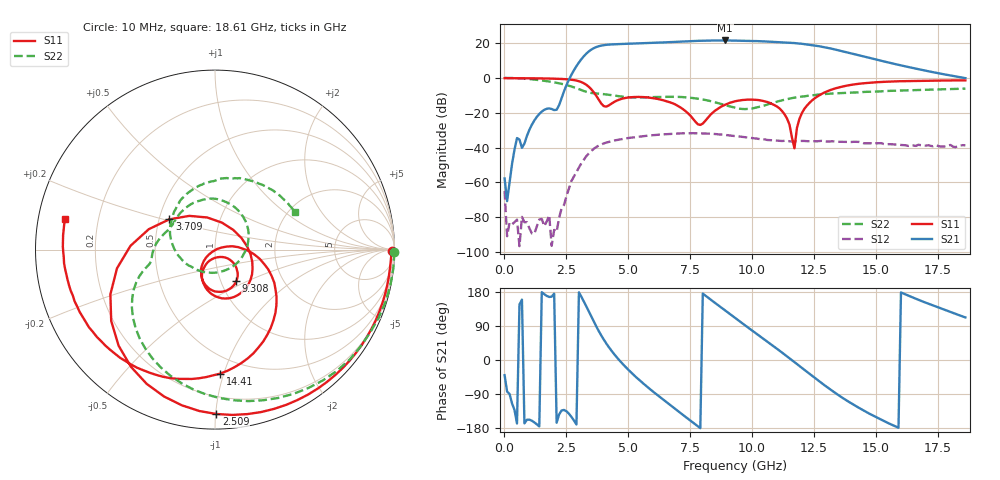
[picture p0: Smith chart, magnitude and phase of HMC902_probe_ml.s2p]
! Hittite Microwave Corporation
! 20 Alpha Road
! Chelmsford, MA 01824
! http://www.hittite.com
! Tel: 978-250-3343
! Fax: 978-250-3373
! Device:  HMC902
! Description: GaAs HEMT MMIC Low Noise Amplifier
! Frequency:  5.00 - 10.00 GHz
! Package:  DIE
! Ports:  2 RF, 4 DC
!  Pad 1 = RF in  = Port 1
!  Pad 2 = Vdd1
!  Pad 3 = Vdd2
!  Pad 4 = RF Out = Port 2
!  Pad 5 = Vgg2 (Optional)
!  Pad 6 = Vgg1 (Optional)
! Voltages:  Vdd = Vdd1 = Vdd2 =  3.50 Volts
!  Idd = Idd1 + Idd2 =  90.03 mA
!  Vgg = Vgg1 = Vgg2 =  Not Used
!  Igg = Igg1 + Igg2 =  Not Used
! Data:  The device was measured using G-S-G Probes on a microstrip
!  alumina (5mil thick) launch with 1 mil wirebonds of approximately 20 mils
!  in length to the RF ports. The microstrip launch is 280 mils long.
!  Data was collected using an calibrated network analyzer.
!  The reference plane is the pads on the microstrip launch.
! Misc:  Validation Unit 3
! Date Measured:  2010-03-25
! Date:  2011-10-27  MJV
! Note:
!  Hittite supplies this data as a sample of measured data at the package pin for
!  for this package product.  Your particular data for this product may vary.
!  Data was taken at 25 degrees C.
!  Hittite reserves the right to change this data at anytime.
!  Data was taken at 25 degrees C.
# GHZ S DB R 50.0
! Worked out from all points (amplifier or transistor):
!   187 points, 10 MHz to 18.61 GHz, reference 50 ohm
!   highest |S21| = 21.5 dB at 8.908 GHz (marker M1)
!   |S21| within 3 dB of that: 3.898 GHz to 12.56 GHz (8.66 GHz wide, 105 % of centre)
!   unconditionally stable (mu >= 1): 14.81 MHz to end of sweep
!   at 3.109 GHz: K = 13.53, MAG = 15.6 dB, |S12| = -49.0 dB
!   at 9.308 GHz: K = 2.00, MAG = 21.7 dB, |S12| = -33.4 dB
!   at 18.61 GHz: K = 8.75, MAG = 6.9 dB, |S12| = -38.7 dB
!   S11 on the Smith chart (normalised r, x): 10 MHz: open; 2.509 GHz: 0.09, -1.00; 3.709 GHz: 0.57, +0.21; 9.308 GHz: 1.18, -0.44; 14.41 GHz: 0.37, -0.97; 18.61 GHz: 0.08, +0.10
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0.01  -0.13 -0.4  -57.78 -40.0  -64.95 16.2  0.00 -0.8
2.50938  -0.76 -89.6  -4.05 -135.5  -67.76 -13.3  -4.11 -135.2
3.10923  -2.40 -135.1  10.79 166.8  -49.00 -77.6  -7.00 -160.6
3.40915  -5.10 -169.2  15.24 127.9  -43.35 -113.1  -8.38 -166.8
3.70908  -10.30 146.5  17.74 88.7  -39.69 -148.2  -8.95 -172.0
4.20895  -15.86 23.5  19.14 34.6  -36.77 162.4  -9.66 173.9
4.70883  -12.11 -33.6  19.49 -5.8  -35.25 126.1  -10.66 161.3
5.50863  -10.95 -71.3  19.86 -56.5  -33.61 81.0  -11.21 144.8
6.20845  -12.14 -94.9  20.27 -94.2  -32.63 47.3  -10.93 125.0
6.90828  -15.32 -115.2  20.77 -129.8  -32.02 16.8  -10.87 99.8
7.70808  -25.13 -107.0  21.25 -169.8  -31.78 -17.2  -11.73 63.7
8.30793  -21.31 -34.8  21.47 160.3  -32.06 -41.1  -13.29 31.7
8.90778  -15.43 -43.4  21.53 130.6  -32.76 -63.4  -15.69 -6.7
9.30768  -13.44 -56.1  21.45 111.1  -33.42 -76.3  -17.14 -38.9
10.10748  -12.57 -86.4  21.21 72.5  -34.71 -98.8  -17.21 -114.2
11.00725  -16.49 -120.9  20.66 29.2  -36.11 -117.5  -13.62 -171.4
11.70708  -40.45 14.2  20.03 -5.7  -36.23 -130.0  -11.32 157.7
12.4069  -13.05 -7.3  18.84 -41.3  -36.34 -148.3  -10.04 134.0
13.2067  -6.70 -42.3  16.80 -80.2  -36.41 -169.0  -9.02 112.2
14.4064  -3.20 -87.6  12.65 -129.8  -37.05 157.4  -8.23 88.7
15.50613  -2.14 -120.6  8.86 -167.0  -38.06 134.4  -7.46 69.3
18.60535  -1.40 168.4  -0.12 112.3  -38.74 70.9  -6.16 25.2
